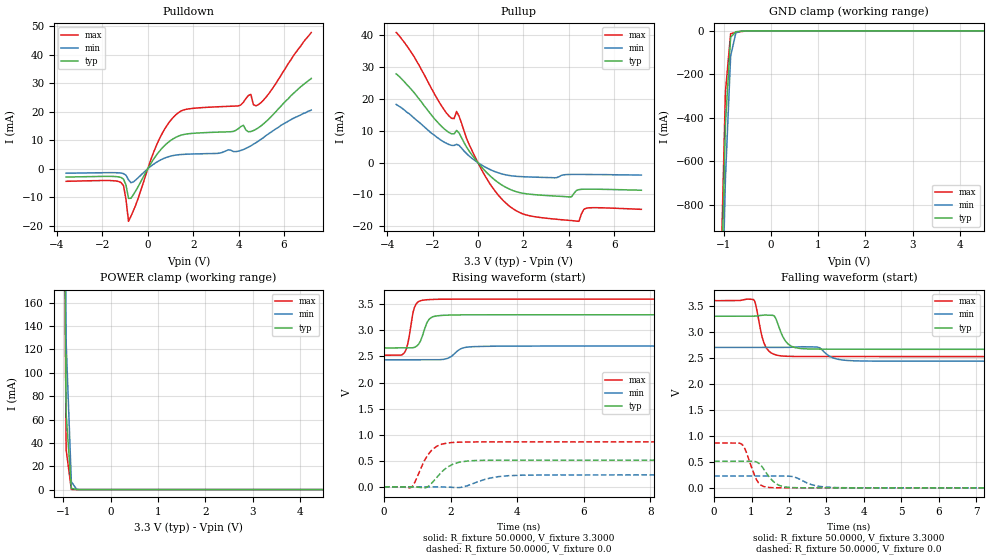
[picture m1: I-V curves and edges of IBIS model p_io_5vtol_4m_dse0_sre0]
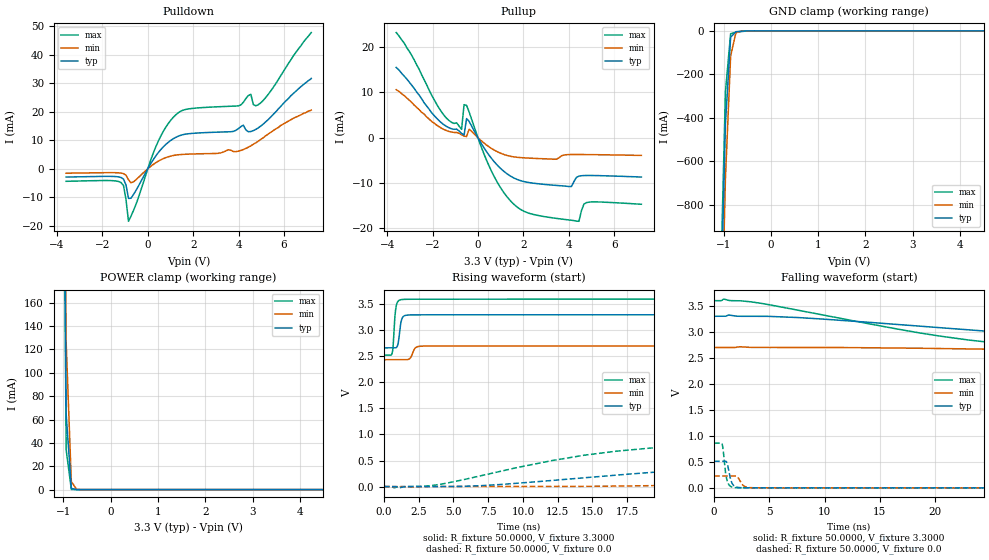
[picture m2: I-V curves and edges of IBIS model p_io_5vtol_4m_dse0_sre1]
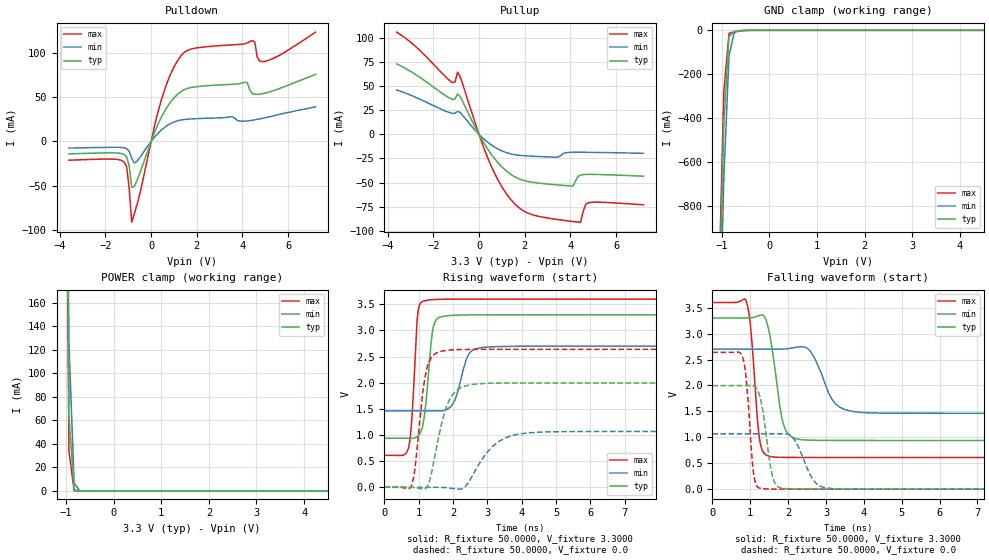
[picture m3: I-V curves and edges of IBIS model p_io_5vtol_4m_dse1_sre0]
| IBIS file nevis_64lqfp_normal.ibs generated by Daphne version: 2018.03.27
[IBIS Ver]   5.0
[Comment Char]   |_char
[File Name]   nevis_64lqfp_normal.ibs
[File Rev]   1
[Date]   Tue Nov  6 16:55:37 2018
[Source]   NXP Viper 2018.03.27
[Notes]
[Disclaimer] IMPORTANT NOTICE
  This information is provided on an AS IS basis and without warranty.
  IN NO EVENT SHALL NXP BE LIABLE FOR INCIDENTAL OR CONSEQUENTIAL
  DAMAGES ARISING FROM USE OF THIS INFORMATION. THIS DISCLAIMER OF
  WARRANTY EXTENDS TO THE USER OF THE INFORMATION, AND TO THEIR CUSTOMERS
  OR USERS OF PRODUCTS  AND IS IN LIEU OF ALL WARRANTIES WHETHER EXPRESS,
  IMPLIED, OR STATUTORY, INCLUDING IMPLIED WARRANTIES OF MERCHANTABILITY
  OR FITNESS FOR PARTICULAR PURPOSE.
  NXP does not represent or warrant that the information furnished
  hereunder is free of infringement of any third party patents,
  copyrights, trade secrets, or other intellectual property rights.
  NXP does not represent or warrant that the information is free of
  defect, or that it meets any particular standard, requirements or need
  of the user of the infomation or their customers.
  NXP reserves the right to change the information in this file
  without notice.
   http://www.nxp.com
[Copyright]   (C) Copyright NXP 2004 - 2018, All Rights Reserved.
|   NEVIS:64LQFP
[Component]   NEVIS:64LQFP
[Manufacturer]   NXP
[Package]
| variable   typ   min   max
R_pkg   0.18765   0.10323   0.21695
L_pkg   3.480e-09   3.024e-09   4.048e-09
C_pkg   4.328e-13   3.597e-13   5.462e-13
[Pin] signal_name   model_name   R_pin   L_pin   C_pin
1   TCK   p_io_5vtol_4m   0.20456   3.984e-09 4.456e-13
2   RESETB   p_vpp_5vtol_4m   0.10323   3.039e-09 5.462e-13
3   GPIOC0   p_io_5vtol_4m   0.18188   3.579e-09 5.125e-13
4   GPIOC1   p_io_5vtol_4m   0.17477   3.449e-09 4.197e-13
5   GPIOC2   p_io_5vtol_4m   0.17199   3.328e-09 4.057e-13
6   GPIOF8   p_io_5vtol_4m   0.1723   3.305e-09 3.675e-13
7   GPIOC3   p_io_5vtol_4m   0.17684   3.425e-09 4.342e-13
8   GPIOC4   p_io_5vtol_4m   0.17579   3.259e-09 3.771e-13
9   GPIOA7   p_io_5vtol_4m   0.1766   3.270e-09 3.648e-13
10   GPIOA6   p_io_5vtol_4m   0.17469   3.370e-09 3.597e-13
11   GPIOA5   p_io_5vtol_4m   0.17299   3.312e-09 3.848e-13
12   GPIOA4   p_io_5vtol_4m   0.17384   3.353e-09 4.083e-13
13   GPIOA0   p_io_5vtol_4m   0.17737   3.491e-09 4.216e-13
14   GPIOA1   p_io_5vtol_4m   0.18461   3.630e-09 4.562e-13
15   GPIOA2   p_io_5vtol_4m   0.19478   3.814e-09 5.013e-13
16   GPIOA3   p_io_5vtol_4m   0.20733   4.048e-09 4.586e-13
17   GPIOB7   p_io_5vtol_4m   0.20924   3.983e-09 4.401e-13
18   GPIOC5   p_io_5vtol_4m   0.10594   3.024e-09 5.247e-13
19   GPIOB6   p_io_5vtol_4m   0.19031   3.559e-09 4.944e-13
20   GPIOB5   p_io_5vtol_4m   0.18832   3.408e-09 4.217e-13
21   GPIOB4   p_io_5vtol_4m   0.19481   3.097e-09 4.139e-13
22   VDDA   POWER   NA   NA   NA
23   VSSA   GND   NA   NA   NA
24   GPIOB0   p_io_5vtol_4m   0.20499   3.148e-09 4.021e-13
25   GPIOB1   p_io_5vtol_4m   0.20867   3.139e-09 4.022e-13
26   VDD   POWER   NA   NA   NA
27   GPIOB2   p_io_5vtol_4m   0.21695   3.397e-09 3.938e-13
28   GPIOB3   p_io_5vtol_4m   0.20181   3.179e-09 4.053e-13
29   VDD33   POWER   NA   NA   NA
30   VSS   GND   NA   NA   NA
31   GPIOC6   p_io_5vtol_4m   0.20223   3.559e-09 4.815e-13
32   GPIOC7   p_io_5vtol_4m   0.20941   3.890e-09 4.421e-13
33   GPIOC8   p_io_5vtol_4m   0.20238   3.900e-09 4.381e-13
34   GPIOC9   p_io_5vtol_4m   0.18996   3.674e-09 4.850e-13
35   GPIOC10   p_io_5vtol_4m   0.18024   3.492e-09 4.400e-13
36   GPIOF0   p_io_5vtol_4m   0.17364   3.367e-09 3.978e-13
37   GPIOC11   p_io_5vtol_4m   0.17763   3.335e-09 3.915e-13
38   GPIOC12   p_io_5vtol_4m   0.17471   3.255e-09 3.726e-13
39   GPIOF2   p_io_5vtol_4m   0.17479   3.285e-09 3.730e-13
40   GPIOF3   p_io_5vtol_4m   0.17558   3.122e-09 3.751e-13
41   GPIOF4   p_io_5vtol_4m   0.1783   3.099e-09 3.845e-13
42   GPIOF5   p_io_5vtol_4m   0.18425   3.161e-09 4.158e-13
43   VSS   GND   NA   NA   NA
44   VDD33   POWER   NA   NA   NA
45   GPIOE0   p_io_5vtol_4m   0.18986   3.116e-09 4.169e-13
46   GPIOE1   p_io_5vtol_4m   0.19417   3.542e-09 4.935e-13
47   GPIOE2   p_io_5vtol_4m   0.19022   3.627e-09 4.739e-13
48   GPIOE3   p_io_5vtol_4m   0.20246   3.876e-09 4.382e-13
49   GPIOC13   p_io_5vtol_4m   0.20528   4.014e-09 4.475e-13
50   GPIOF1   p_io_5vtol_4m   0.1965   3.833e-09 4.884e-13
51   GPIOE4   p_io_5vtol_4m   0.2004   3.843e-09 4.592e-13
52   GPIOE5   p_io_5vtol_4m   0.19457   3.717e-09 4.386e-13
53   GPIOE6   p_io_5vtol_4m   0.19219   3.582e-09 4.273e-13
54   GPIOE7   p_io_5vtol_4m   0.19237   3.536e-09 3.947e-13
55   GPIOC14   p_io_5vtol_4m   0.19532   3.570e-09 3.956e-13
56   GPIOC15   p_io_5vtol_4m   0.19877   3.342e-09 3.979e-13
57   VDD   POWER   NA   NA   NA
58   GPIOF6   p_io_5vtol_4m   0.20225   3.248e-09 4.630e-13
59   GPIOF7   p_io_5vtol_4m   0.1991   3.203e-09 3.918e-13
60   VDD33   POWER   NA   NA   NA
61   VSS   GND   NA   NA   NA
62   TDO   p_io_5vtol_4m   0.19991   3.386e-09 5.235e-13
63   TMS   p_io_5vtol_4m   0.20172   3.751e-09 5.036e-13
64   TDI   p_io_5vtol_4m   0.21043   4.005e-09 4.589e-13
65   NC   NC   NA   NA   NA
[Pin Mapping]   pulldown_ref   pullup_ref
1   NC   NC
2   NC   NC
3   NC   NC
4   NC   NC
5   NC   NC
6   NC   NC
7   NC   NC
8   NC   NC
9   NC   NC
10   NC   NC
11   NC   NC
12   NC   NC
13   NC   NC
14   NC   NC
15   NC   NC
16   NC   NC
17   NC   NC
18   NC   NC
19   NC   NC
20   NC   NC
21   NC   NC
22   NC   VDDA
23   VSSA   NC
24   NC   NC
25   NC   NC
26   NC   VDD
27   NC   NC
28   NC   NC
29   NC   VDD33
30   VSS   NC
31   NC   NC
32   NC   NC
33   NC   NC
34   NC   NC
35   NC   NC
36   NC   NC
37   NC   NC
38   NC   NC
39   NC   NC
40   NC   NC
41   NC   NC
42   NC   NC
43   VSS   NC
44   NC   VDD33
45   NC   NC
46   NC   NC
47   NC   NC
48   NC   NC
49   NC   NC
50   NC   NC
51   NC   NC
52   NC   NC
53   NC   NC
54   NC   NC
55   NC   NC
56   NC   NC
57   NC   VDD
58   NC   NC
59   NC   NC
60   NC   VDD33
61   VSS   NC
62   NC   NC
63   NC   NC
64   NC   NC
65   NC   NC
|*   Model Selector   *
[Model Selector] p_io_5vtol_4m
p_io_5vtol_4m_dse1_sre0   io, full drive mode without slew rate
p_io_5vtol_4m_dse1_sre1   io, full drive mode with slew rate
p_io_5vtol_4m_dse0_sre0   io, low drive mode without slew rate
p_io_5vtol_4m_dse0_sre1   io, low drive mode with slew rate
| End [Component] NEVIS:64LQFP
| Models and submodels in the file (5): p_io_5vtol_4m_dse0_sre0 (I/O), p_io_5vtol_4m_dse0_sre1 (I/O), p_io_5vtol_4m_dse1_sre0 (I/O), p_io_5vtol_4m_dse1_sre1 (I/O), p_vpp_5vtol_4m (I/O_open_drain)
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[Model] p_io_5vtol_4m_dse0_sre0
|   Model p_io_5vtol_4m_dse0_sre0
| Library cells for typ/min/max conditions are connected as defined below:
|  pad - External Pad
|  ipp_do - Core Input
|  ipp_obe - Output Buffer Enable
|  esd_boost - vdd_s_3v
|  esd_bus - vdd_s_3v
|  ipp_ame - vss_s_lv
|  ipp_dse - vss_s_lv
|  ipp_ina40a_5vtol - NC
|  ipp_ina40b_5vtol - NC
|  ipp_ina_5vtol - NC
|  ipp_ina_mux_3v - NC
|  ipp_ind - NC
|  ipp_ind_3v - NC
|  ipp_pue - vss_s_lv
|  ipp_sre - vss_s_lv
|  tie_3v - vdd_s_3v
|  tie_hi - vdd_s_lv
|  vbuf_3v - vdd_s_3v
|  vdd_bulk_lv - vdd_s_lv
|  vdd_s_3v - vdd_s_3v
|  vdd_s_lv - vdd_s_lv
|  vss_bulk - vss_s_3v
|  vss_s_3v - vss_s_3v
|  vss_s_lv - vss_s_lv
| All other pins connected to ground
Model_type I/O
Polarity   Non-Inverting
Enable   Active-High
Vinl =   1.1550V
Vinh =   2.3100V
Vmeas =  1.6500V
Cref =   25.0000pF
Rref =   0.5000k
Vref =   0.0V
C_comp   2.7442pF   2.6088pF   2.9166pF
[Temperature Range]   25.0000   0.1250k   -40.0000
[Voltage Range]   3.3000V   2.7000V   3.6000V
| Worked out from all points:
|   slope of the pulldown table from 0 to 0.495 V, typ, clamps not added: 82.8 ohm
|   slope of the pullup table from 0 to 0.495 V, typ, clamps not added: 127 ohm
|   GND clamp passes 1 mA (typ) near -0.56 V on its own axis
|   POWER clamp passes 1 mA (typ) near -0.82 V on its own axis
|   rising waveform, R_fixture 50.0000, V_fixture 3.3000: 20-80 % time 220ps typ, 318ps min, 177ps max; typ from 2.66 V to 3.3 V
|   rising waveform, R_fixture 50.0000, V_fixture 0.0: 20-80 % time 520ps typ, 708ps min, 427ps max; typ from 0 V to 0.512 V
|   falling waveform, R_fixture 50.0000, V_fixture 3.3000: 20-80 % time 253ps typ, 333ps min, 210ps max; typ from 3.3 V to 2.66 V
|   falling waveform, R_fixture 50.0000, V_fixture 0.0: 20-80 % time 337ps typ, 455ps min, 264ps max; typ from 0.512 V to 0 V
[Pulldown]
|Voltage   I(typ)   I(min)   I(max)
-3.6V     -2.92mA    -1.56mA    -4.41mA
-1.18V    -3.075mA   -1.514mA   -4.85mA
-1.07V    -3.642mA   -1.711mA   -5.917mA
-850mV    -10.41mA   -3.881mA   -18.45mA
360mV     4.579mA    2.156mA    7.833mA
1.13V     10.56mA    4.658mA    18.11mA
1.79V     12.28mA    5.123mA    21mA
3.99V     14.08mA    6.16mA     22.06mA
4.54V     13.07mA    8.03mA     26.11mA
4.65V     13.38mA    8.6mA      22.52mA
4.87V     14.37mA    9.7mA      22.49mA
7.2V      31.7mA     20.6mA     47.8mA
[Pullup]
|Voltage   I(typ)   I(min)   I(max)
-3.6V     27.9mA     18.3mA     40.9mA
-2.81V    22mA       14mA       33.3mA
-1.38V    10.01mA    6.04mA     15.54mA
-1.05V    9.045mA    5.403mA    13.85mA
-940mV    10.12mA    5.768mA    16.08mA
-390mV    3.678mA    2.088mA    5.744mA
270mV     -2.258mA   -1.197mA   -3.638mA
1.48V     -8.613mA   -4.152mA   -14.19mA
4.01V     -10.78mA   -3.728mA   -18.16mA
4.45V     -8.487mA   -3.709mA   -18.45mA
4.78V     -8.342mA   -3.73mA    -14.33mA
7.2V      -8.69mA    -3.91mA    -14.69mA
[GND_clamp]
|Voltage   I(typ)   I(min)   I(max)
-3.6V     -31.15A    -31.13A    -31.21A
-1.07V    -1.387A    -1.641A    -1.238A
-960mV    -429.3mA   -680.2mA   -281.1mA
-850mV    -29.75mA   -116.1mA   -13.24mA
-740mV    -4.234mA   -9.703mA   -7.092mA
-630mV    -1.925mA   -1.63mA    -3.569mA
-410mV    -31.96uA   -64.36uA   -35uA
7.2V      0A         0A         0A
[POWER_clamp]
|Voltage   I(typ)   I(min)   I(max)
-3.6V     31.35A     31.03A     31.61A
-1.05V    682.2mA    740.4mA    662.9mA
-940mV    65.1mA     126.6mA    34.32mA
-830mV    1.105mA    6.829mA    165.4uA
-720mV    15.33uA    281.3uA    694.4nA
-610mV    212.1nA    11.41uA    2.964nA
7.2V      0A         0A         0A
[Ramp]
| variable   typ   min   max
dV/dt_r  0.3070/0.5203n   0.1368/0.7078n   0.5174/0.4265n
dV/dt_f  0.3816/0.2526n   0.1581/0.3329n   0.6454/0.2102n
R_load = 50.0000
[Rising Waveform]
R_fixture= 50.0000
V_fixture= 3.3000
V_fixture_min= 2.7000
V_fixture_max= 3.6000
|time   V(typ)   V(min)   V(max)
0s        2.664V     2.436V     2.524V
610.3ps   2.664V     2.436V     2.569V
714.5ps   2.664V     2.436V     2.741V
910.9ps   2.675V     2.436V     3.431V
1.094ns   2.792V     2.437V     3.568V
1.273ns   3.119V     2.437V     3.588V
1.552ns   3.276V     2.437V     3.596V
2.35ns    3.298V     2.659V     3.599V
2.979ns   3.3V       2.694V     3.599V
20ns      3.3V       2.7V       3.6V
[Rising Waveform]
R_fixture= 50.0000
V_fixture= 0.0
V_fixture_min= 0.0
V_fixture_max= 0.0
|time   V(typ)   V(min)   V(max)
0s        1.096nV    96.66nV    914.3pV
817.3ps   -174.2uV   1.791uV    -11.85mV
1.238ns   -20.09mV   132uV      527.3mV
1.432ns   68.46mV    364.3uV    703.1mV
1.774ns   310.6mV    -2.683mV   823mV
2.042ns   424.3mV    -10.1mV    850.1mV
2.694ns   503.4mV    66.34mV    860.8mV
3.192ns   509.9mV    168.5mV    861.5mV
4.049ns   511.3mV    221.6mV    861.7mV
20ns      511.7mV    228.1mV    862.3mV
[Falling Waveform]
R_fixture= 50.0000
V_fixture= 3.3000
V_fixture_min= 2.7000
V_fixture_max= 3.6000
|time   V(typ)   V(min)   V(max)
0s        3.3V       2.7V       3.6V
1.056ns   3.301V     2.7V       3.62V
1.285ns   3.321V     2.7V       2.894V
1.39ns    3.322V     2.7V       2.695V
1.614ns   3.301V     2.7V       2.565V
1.898ns   2.83V      2.7V       2.531V
2.744ns   2.668V     2.71V      2.525V
3.178ns   2.667V     2.499V     2.525V
3.812ns   2.665V     2.441V     2.525V
20ns      2.664V     2.436V     2.524V
[Falling Waveform]
R_fixture= 50.0000
V_fixture= 0.0
V_fixture_min= 0.0
V_fixture_max= 0.0
|time   V(typ)   V(min)   V(max)
0s        511.8mV    228.1mV    862.4mV
740.7ps   511.8mV    228.1mV    838mV
824.6ps   511.7mV    228.1mV    750.7mV
1.166ns   486.7mV    228.1mV    119mV
1.481ns   202.1mV    228.1mV    6.302mV
1.652ns   81.2mV     228mV      2.01mV
1.911ns   16.02mV    227.7mV    767.9uV
2.752ns   448uV      36.41mV    432.9uV
3.473ns   288.4uV    2.353mV    359uV
20ns      60.38uV    38.43uV    87.29uV
[Model] p_io_5vtol_4m_dse0_sre1
|   Model p_io_5vtol_4m_dse0_sre1
| Library cells for typ/min/max conditions are connected as defined below:
|  pad - External Pad
|  ipp_do - Core Input
|  ipp_obe - Output Buffer Enable
|  esd_boost - vdd_s_3v
|  esd_bus - vdd_s_3v
|  ipp_ame - vss_s_lv
|  ipp_dse - vss_s_lv
|  ipp_ina40a_5vtol - NC
|  ipp_ina40b_5vtol - NC
|  ipp_ina_5vtol - NC
|  ipp_ina_mux_3v - NC
|  ipp_ind - NC
|  ipp_ind_3v - NC
|  ipp_pue - vss_s_lv
|  ipp_sre - vdd_s_lv
|  tie_3v - vdd_s_3v
|  tie_hi - vdd_s_lv
|  vbuf_3v - vdd_s_3v
|  vdd_bulk_lv - vdd_s_lv
|  vdd_s_3v - vdd_s_3v
|  vdd_s_lv - vdd_s_lv
|  vss_bulk - vss_s_3v
|  vss_s_3v - vss_s_3v
|  vss_s_lv - vss_s_lv
| All other pins connected to ground
Model_type I/O
Polarity   Non-Inverting
Enable   Active-High
Vinl =   1.1550V
Vinh =   2.3100V
Vmeas =  1.6500V
Cref =   25.0000pF
Rref =   0.5000k
Vref =   0.0V
C_comp   2.7442pF   2.6088pF   2.9166pF
[Temperature Range]   25.0000   0.1250k   -40.0000
[Voltage Range]   3.3000V   2.7000V   3.6000V
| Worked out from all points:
|   slope of the pulldown table from 0 to 0.495 V, typ, clamps not added: 82.8 ohm
|   slope of the pullup table from 0 to 0.495 V, typ, clamps not added: 127 ohm
|   GND clamp passes 1 mA (typ) near -0.56 V on its own axis
|   POWER clamp passes 1 mA (typ) near -0.82 V on its own axis
|   rising waveform, R_fixture 50.0000, V_fixture 3.3000: 20-80 % time 192ps typ, 268ps min, 163ps max; typ from 2.66 V to 3.3 V
|   rising waveform, R_fixture 50.0000, V_fixture 0.0: 20-80 % time 17.3ns typ, 32.4ns min, 10.8ns max; typ from 0 V to 0.512 V
|   falling waveform, R_fixture 50.0000, V_fixture 3.3000: 20-80 % time 29.9ns typ, 51ns min, 19.5ns max; typ from 3.3 V to 2.66 V
|   falling waveform, R_fixture 50.0000, V_fixture 0.0: 20-80 % time 342ps typ, 422ps min, 300ps max; typ from 0.512 V to 0 V
[Pulldown]
|Voltage   I(typ)   I(min)   I(max)
-3.6V     -2.92mA    -1.56mA    -4.41mA
-1.18V    -3.075mA   -1.514mA   -4.85mA
-1.07V    -3.642mA   -1.711mA   -5.917mA
-850mV    -10.41mA   -3.881mA   -18.45mA
360mV     4.579mA    2.156mA    7.833mA
1.13V     10.56mA    4.658mA    18.11mA
1.79V     12.28mA    5.123mA    21mA
3.99V     14.08mA    6.16mA     22.06mA
4.54V     13.07mA    8.03mA     26.11mA
4.65V     13.38mA    8.6mA      22.52mA
4.87V     14.37mA    9.7mA      22.49mA
7.2V      31.7mA     20.6mA     47.8mA
[Pullup]
|Voltage   I(typ)   I(min)   I(max)
-3.6V     15.5mA     10.6mA     23.2mA
-1.38V    2.47mA     1.56mA     4.28mA
-720mV    935.3uA    641.5uA    1.84mA
-610mV    580.7uA    348.6uA    7.293mA
-500mV    4.215mA    257.3uA    7.125mA
-390mV    3.605mA    1.85mA     5.718mA
710mV     -5.257mA   -2.715mA   -8.512mA
1.81V     -9.375mA   -4.366mA   -15.61mA
4.12V     -10.77mA   -3.714mA   -18.22mA
4.45V     -8.487mA   -3.709mA   -18.45mA
4.78V     -8.342mA   -3.73mA    -14.33mA
7.2V      -8.69mA    -3.91mA    -14.69mA
[GND_clamp]
|Voltage   I(typ)   I(min)   I(max)
-3.6V     -31.15A    -31.13A    -31.21A
-1.07V    -1.387A    -1.641A    -1.238A
-960mV    -429.3mA   -680.2mA   -281.1mA
-850mV    -29.75mA   -116.1mA   -13.24mA
-740mV    -4.234mA   -9.703mA   -7.092mA
-630mV    -1.925mA   -1.63mA    -3.569mA
-410mV    -31.96uA   -64.36uA   -35uA
7.2V      0A         0A         0A
[POWER_clamp]
|Voltage   I(typ)   I(min)   I(max)
-3.6V     31.35A     31.03A     31.61A
-1.05V    682.2mA    740.4mA    662.9mA
-940mV    65.1mA     126.6mA    34.32mA
-830mV    1.105mA    6.829mA    165.4uA
-720mV    15.33uA    281.3uA    694.4nA
-610mV    212.1nA    11.41uA    2.964nA
7.2V      0A         0A         0A
[Ramp]
| variable   typ   min   max
dV/dt_r  0.3071/17.2926n   0.1369/32.3674n   0.5175/10.7611n
dV/dt_f  0.3817/29.8719n   0.1576/51.0200n   0.6456/19.5314n
R_load = 50.0000
[Rising Waveform]
R_fixture= 50.0000
V_fixture= 3.3000
V_fixture_min= 2.7000
V_fixture_max= 3.6000
|time   V(typ)   V(min)   V(max)
0s        2.664V     2.437V     2.524V
605.3ps   2.664V     2.437V     2.579V
657.9ps   2.664V     2.437V     2.693V
807.7ps   2.664V     2.437V     3.325V
923.6ps   2.679V     2.436V     3.511V
1.276ns   3.209V     2.437V     3.592V
1.646ns   3.293V     2.437V     3.597V
2.341ns   3.298V     2.679V     3.598V
3.739ns   3.299V     2.699V     3.598V
250ns     3.3V       2.7V       3.6V
[Rising Waveform]
R_fixture= 50.0000
V_fixture= 0.0
V_fixture_min= 0.0
V_fixture_max= 0.0
|time   V(typ)   V(min)   V(max)
0s        1.096nV    96.66nV    914.3pV
730.2ps   540.1uV    1.417uV    -25.29mV
3.533ns   -267.8uV   -118.1uV   22.43mV
11.84ns   111.3mV    1.042mV    487mV
16.8ns    222mV      9.094mV    681.3mV
24.08ns   354mV      38.46mV    807.6mV
31.02ns   430.3mV    75.05mV    845.8mV
49.75ns   501.2mV    160.4mV    861.8mV
86.96ns   511.7mV    219.4mV    862.5mV
250ns     511.8mV    228.1mV    862.5mV
[Falling Waveform]
R_fixture= 50.0000
V_fixture= 3.3000
V_fixture_min= 2.7000
V_fixture_max= 3.6000
|time   V(typ)   V(min)   V(max)
0s        3.3V       2.7V       3.6V
896.8ps   3.3V       2.7V       3.63V
3.769ns   3.3V       2.7V       3.565V
18.49ns   3.112V     2.686V     2.984V
25.66ns   2.998V     2.664V     2.78V
33.75ns   2.887V     2.635V     2.66V
43.81ns   2.796V     2.595V     2.594V
65.21ns   2.714V     2.521V     2.543V
96.83ns   2.677V     2.472V     2.527V
250ns     2.664V     2.437V     2.524V
[Falling Waveform]
R_fixture= 50.0000
V_fixture= 0.0
V_fixture_min= 0.0
V_fixture_max= 0.0
|time   V(typ)   V(min)   V(max)
0s        511.8mV    228.1mV    862.4mV
711.3ps   511.8mV    228.1mV    851.3mV
813.8ps   511.8mV    228.1mV    743.1mV
1.045ns   511.3mV    228.1mV    281.6mV
1.18ns    474mV      228.1mV    137.9mV
1.57ns    116.7mV    228mV      19.01mV
2.147ns   7.963mV    204.4mV    2.261mV
2.747ns   1.249mV    29.86mV    1.357mV
3.983ns   641.3uV    486.1uV    1mV
250ns     26.94nV    927.1nV    8.795nV
[Model] p_io_5vtol_4m_dse1_sre0
|   Model p_io_5vtol_4m_dse1_sre0
| Library cells for typ/min/max conditions are connected as defined below:
|  pad - External Pad
|  ipp_do - Core Input
|  ipp_obe - Output Buffer Enable
|  esd_boost - vdd_s_3v
|  esd_bus - vdd_s_3v
|  ipp_ame - vss_s_lv
|  ipp_dse - vdd_s_lv
|  ipp_ina40a_5vtol - NC
|  ipp_ina40b_5vtol - NC
|  ipp_ina_5vtol - NC
|  ipp_ina_mux_3v - NC
|  ipp_ind - NC
|  ipp_ind_3v - NC
|  ipp_pue - vss_s_lv
|  ipp_sre - vss_s_lv
|  tie_3v - vdd_s_3v
|  tie_hi - vdd_s_lv
|  vbuf_3v - vdd_s_3v
|  vdd_bulk_lv - vdd_s_lv
|  vdd_s_3v - vdd_s_3v
|  vdd_s_lv - vdd_s_lv
|  vss_bulk - vss_s_3v
|  vss_s_3v - vss_s_3v
|  vss_s_lv - vss_s_lv
| All other pins connected to ground
Model_type I/O
Polarity   Non-Inverting
Enable   Active-High
Vinl =   1.1550V
Vinh =   2.3100V
Vmeas =  1.6500V
Cref =   25.0000pF
Rref =   0.5000k
Vref =   0.0V
C_comp   2.7442pF   2.6088pF   2.9166pF
[Temperature Range]   25.0000   0.1250k   -40.0000
[Voltage Range]   3.3000V   2.7000V   3.6000V
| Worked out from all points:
|   slope of the pulldown table from 0 to 0.495 V, typ, clamps not added: 16.7 ohm
|   slope of the pullup table from 0 to 0.495 V, typ, clamps not added: 25.7 ohm
|   GND clamp passes 1 mA (typ) near -0.56 V on its own axis
|   POWER clamp passes 1 mA (typ) near -0.82 V on its own axis
|   rising waveform, R_fixture 50.0000, V_fixture 3.3000: 20-80 % time 198ps typ, 316ps min, 148ps max; typ from 0.938 V to 3.3 V
|   rising waveform, R_fixture 50.0000, V_fixture 0.0: 20-80 % time 433ps typ, 731ps min, 266ps max; typ from 0 V to 2 V
|   falling waveform, R_fixture 50.0000, V_fixture 3.3000: 20-80 % time 273ps typ, 438ps min, 181ps max; typ from 3.3 V to 0.939 V
|   falling waveform, R_fixture 50.0000, V_fixture 0.0: 20-80 % time 233ps typ, 387ps min, 161ps max; typ from 2 V to 0 V
[Pulldown]
|Voltage   I(typ)   I(min)   I(max)
-3.6V     -13.95mA   -7.44mA    -21.1mA
-1.18V    -14.7mA    -7.219mA   -23.24mA
-1.07V    -17.36mA   -8.141mA   -28.3mA
-850mV    -51.45mA   -18.95mA   -91.09mA
-630mV    -44.71mA   -22.71mA   -72.44mA
470mV     28.45mA    13.31mA    48.59mA
1.35V     56.89mA    24.4mA     97.86mA
4.1V      66.73mA    22.95mA    110.2mA
4.43V     54.09mA    23.92mA    113.9mA
4.65V     53.15mA    25mA       94.51mA
4.98V     54.48mA    26.7mA     90.35mA
7.2V      75.8mA     39.1mA     123.4mA
[Pullup]
|Voltage   I(typ)   I(min)   I(max)
-3.6V     72.9mA     45.9mA     106mA
-1.16V    36.23mA    21.7mA     53.64mA
-1.05V    36.74mA    21.9mA     54.26mA
-940mV    41.85mA    23.77mA    64.43mA
600mV     -22.66mA   -11.88mA   -36.28mA
1.15V     -36.98mA   -18.56mA   -59.89mA
1.81V     -46.62mA   -21.82mA   -77.16mA
4.12V     -53.36mA   -18.54mA   -90.34mA
4.45V     -42.19mA   -18.52mA   -91.04mA
4.67V     -41.57mA   -18.57mA   -72.57mA
4.78V     -41.5mA    -18.6mA    -70.99mA
7.2V      -43.39mA   -19.66mA   -73.06mA
[GND_clamp]
|Voltage   I(typ)   I(min)   I(max)
-3.6V     -31.15A    -31.13A    -31.21A
-1.07V    -1.387A    -1.641A    -1.238A
-960mV    -429.3mA   -680.2mA   -281.1mA
-850mV    -29.75mA   -116.1mA   -13.24mA
-740mV    -4.234mA   -9.703mA   -7.092mA
-630mV    -1.925mA   -1.63mA    -3.569mA
-410mV    -31.96uA   -64.36uA   -35uA
7.2V      0A         0A         0A
[POWER_clamp]
|Voltage   I(typ)   I(min)   I(max)
-3.6V     31.35A     31.03A     31.61A
-1.05V    682.2mA    740.4mA    662.9mA
-940mV    65.1mA     126.6mA    34.32mA
-830mV    1.105mA    6.829mA    165.4uA
-720mV    15.33uA    281.3uA    694.4nA
-610mV    212.1nA    11.41uA    2.964nA
7.2V      0A         0A         0A
[Ramp]
| variable   typ   min   max
dV/dt_r  1.1975/0.4329n   0.6401/0.7312n   1.5830/0.2663n
dV/dt_f  1.4166/0.2733n   0.7428/0.4382n   1.7935/0.1810n
R_load = 50.0000
[Rising Waveform]
R_fixture= 50.0000
V_fixture= 3.3000
V_fixture_min= 2.7000
V_fixture_max= 3.6000
|time   V(typ)   V(min)   V(max)
0s        938.5mV    1.461V     610.4mV
700.1ps   938.2mV    1.461V     747.1mV
796.4ps   936.7mV    1.461V     1.287V
950.6ps   966.3mV    1.461V     3.178V
1.101ns   1.142V     1.462V     3.551V
1.388ns   2.926V     1.461V     3.588V
1.622ns   3.255V     1.459V     3.595V
1.984ns   3.288V     1.584V     3.598V
2.713ns   3.298V     2.658V     3.599V
10ns      3.3V       2.7V       3.6V
[Rising Waveform]
R_fixture= 50.0000
V_fixture= 0.0
V_fixture_min= 0.0
V_fixture_max= 0.0
|time   V(typ)   V(min)   V(max)
0s        411.9pV    47.82nV    286.1pV
789.5ps   -503.9uV   655.3nV    31.27mV
878.5ps   -6.744mV   -6.775uV   304.7mV
1.188ns   -27.08mV   110.8uV    2.128V
1.538ns   828.6mV    -14.89uV   2.576V
1.891ns   1.669V     -15.27mV   2.625V
2.523ns   1.961V     173.5mV    2.637V
3.139ns   1.99V      774.3mV    2.638V
3.956ns   1.995V     1.021V     2.638V
10ns      1.996V     1.067V     2.638V
[Falling Waveform]
R_fixture= 50.0000
V_fixture= 3.3000
V_fixture_min= 2.7000
V_fixture_max= 3.6000
|time   V(typ)   V(min)   V(max)
0s        3.3V       2.7V       3.6V
897ps     3.3V       2.7V       3.62V
1.012ns   3.302V     2.7V       3.118V
1.248ns   3.352V     2.7V       952.4mV
1.481ns   3.092V     2.7V       637.9mV
1.861ns   1.291V     2.7V       613mV
2.204ns   973.7mV    2.735V     611.7mV
2.551ns   944.9mV    2.689V     611.3mV
3.583ns   939.7mV    1.518V     611mV
10ns      939mV      1.462V     610.8mV
[Falling Waveform]
R_fixture= 50.0000
V_fixture= 0.0
V_fixture_min= 0.0
V_fixture_max= 0.0
|time   V(typ)   V(min)   V(max)
0s        1.996V     1.067V     2.639V
793.2ps   1.996V     1.067V     2.557V
892.4ps   1.996V     1.067V     2.131V
1.088ns   1.992V     1.067V     303.9mV
1.245ns   1.808V     1.067V     21.49mV
1.576ns   285.6mV    1.067V     1.916mV
1.813ns   22.93mV    1.069V     779.9uV
2.113ns   4.177mV    1.006V     534.5uV
2.932ns   535.4uV    34.39mV    380.9uV
10ns      242.2uV    204.3uV    218.8uV
